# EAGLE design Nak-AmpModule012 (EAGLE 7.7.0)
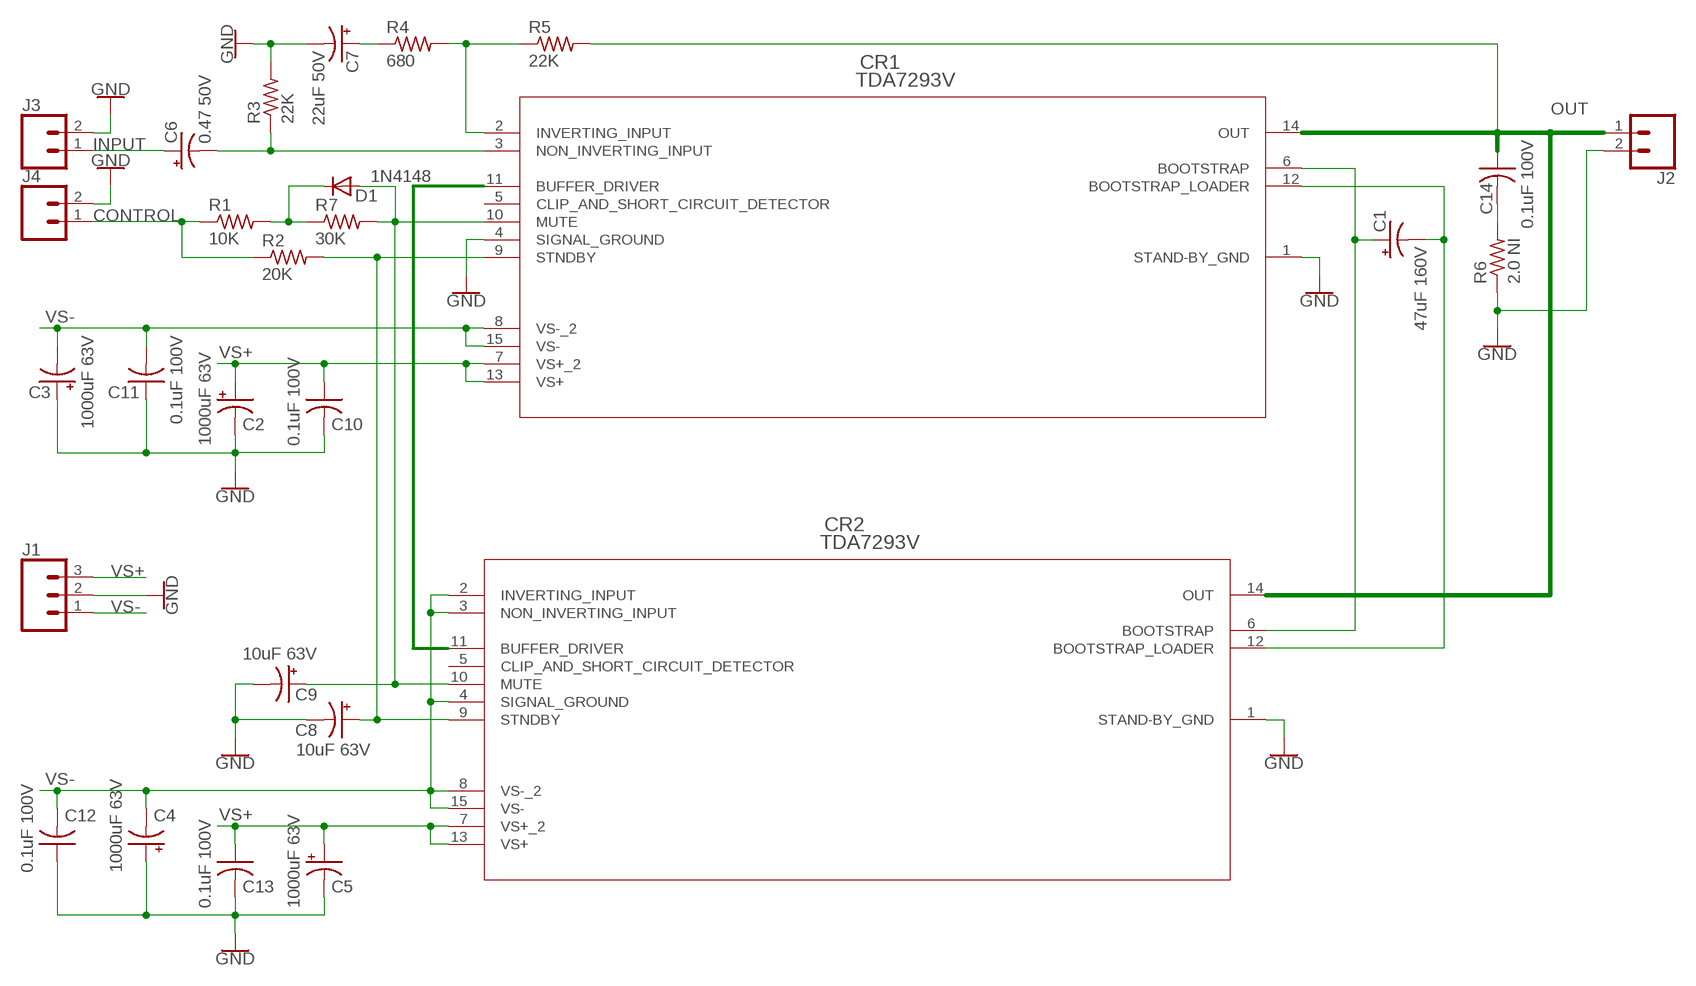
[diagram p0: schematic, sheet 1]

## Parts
C1  47uF 160V  CPOL-USE5-10.5  [E5-10,5]
C2  1000uF 63V  CPOL-USE7.5-16  [E7,5-16]
C3  1000uF 63V  CPOL-USE7.5-16  [E7,5-16]
C4  1000uF 63V  CPOL-USE7.5-16  [E7,5-16]
C5  1000uF 63V  CPOL-USE7.5-16  [E7,5-16]
C6  0.47 50V  CPOL-USE2-5  [E2-5]
C7  22uF 50V  CPOL-USE3.5-8  [E3,5-8]
C8  10uF 63V  CPOL-USE2.5-5  [E2,5-5]
C9  10uF 63V  CPOL-USE2.5-5  [E2,5-5]
C10  0.1uF 100V  C-US025-030X050  [C025-030X050]
C11  0.1uF 100V  C-US025-030X050  [C025-030X050]
C12  0.1uF 100V  C-US025-030X050  [C025-030X050]
C13  0.1uF 100V  C-US025-030X050  [C025-030X050]
C14  0.1uF 100V  C-US025-030X050  [C025-030X050]
CR1  TDA7293V  [MULTIWATT15_V]
CR2  TDA7293V  [MULTIWATT15_V]
D1  1N4148  1N4148DO35-7  [DO35-7]
J1  CONN_03-SCREW-5MM  [SCREWTERMINAL-5MM-3]
J2  CONN_025MM  [SCREWTERMINAL-5MM-2]
J3  CONN_023.5MM  [SCREWTERMINAL-3.5MM-2]
J4  CONN_023.5MM  [SCREWTERMINAL-3.5MM-2]
R1  10K  R-US_0207/10  [0207/10]
R2  20K  R-US_0207/10  [0207/10]
R3  22K  R-US_0204/7  [0204/7]
R4  680  R-US_0207/10  [0207/10]
R5  22K  R-US_0204/7  [0204/7]
R6  2.0 NI  R-US_0411/15  [0411/15]
R7  30K  R-US_0207/10  [0207/10]

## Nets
B-LOADER: C1.- CR1.12(BOOTSTRAP_LOADER) CR2.12(BOOTSTRAP_LOADER)
BOOTSTRAP: C1.+ CR1.6(BOOTSTRAP) CR2.6(BOOTSTRAP)
BUFDRVR: CR1.11(BUFFER_DRIVER) CR2.11(BUFFER_DRIVER)
CONTROL: J4.1 R1.1 R2.1
GND: C2.- C3.+ C4.+ C5.- C7.- C8.- C9.- C10.2 C11.1 C12.1 C13.2 CR1.1(STAND-BY_GND) CR1.4(SIGNAL_GROUND) CR2.1(STAND-BY_GND) J1.2 J2.2 J3.2 J4.2 R3.2 R6.1
INPUT: C6.+ J3.1
INV: CR1.2(INVERTING_INPUT) R4.2 R5.1
MUTE: C9.+ CR1.10(MUTE) CR2.10(MUTE) D1.A R7.2
N$3: C14.2 R6.2
N$11: D1.C R1.2 R7.1
N$16: C7.+ R4.1
NON-INV: C6.- CR1.3(NON_INVERTING_INPUT) R3.1
OUT: C14.1 CR1.14(OUT) CR2.14(OUT) J2.1 R5.2
STNDBY: C8.+ CR1.9(STNDBY) CR2.9(STNDBY) R2.2
VS+: C2.+ C5.+ C10.1 C13.1 CR1.7(VS+_2) CR1.13(VS+) CR2.7(VS+_2) CR2.13(VS+) J1.3
VS-: C3.- C4.- C11.2 C12.2 CR1.8(VS-_2) CR1.15(VS-) CR2.2(INVERTING_INPUT) CR2.3(NON_INVERTING_INPUT) CR2.4(SIGNAL_GROUND) CR2.8(VS-_2) CR2.15(VS-) J1.1
Unconnected: CR1.5(CLIP_AND_SHORT_CIRCUIT_DETECTOR) CR2.5(CLIP_AND_SHORT_CIRCUIT_DETECTOR)

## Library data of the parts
C1 = resistor:CPOL-US: POLARIZED CAPACITOR, American symbol; DESC: 47 µF 160 V Capacitor Radial, 10000 Hrs @ 105C; MFG: Rubycon; PN: 160BXC47MEFC10X20
C2 C3 C5-C9 = resistor:CPOL-US: POLARIZED CAPACITOR, American symbol
C4 = resistor:CPOL-US: POLARIZED CAPACITOR, American symbol; DESC: 1000 µF 63 V Electrolytic Capacitor Radial, 10000 Hrs @ 105°C; MFG: Rubycon; PN: 63ZLJ1000M16X25
C10 C12-C14 = resistor:C-US: CAPACITOR, American symbol
C11 = resistor:C-US: CAPACITOR, American symbol; DESC: 0.1 µF ±10% 100V Ceramic Capacitor X7R Radial; MFG: Vishay; PN: K104K20X7RH53L2
CR1 CR2 = STM-TDA7293V:TDA7293V; BUILT_BY: EMA_UL_Team; MANUFACTURER_PART_NUMBER: TDA7293V; VENDOR: STMicroelectronics
D1 = diode:1N4148: DIODE
J1 = SparkFun-Connectors:CONN_03: Multi connection point. Often used as Generic Header-pin footprint for 0.1 inch spaced/style header connections On any of the 0.1 inch spaced packages, you can populate with these: Break Away Headers - Straight (PRT-00116) Break Away Male Headers - Right Angle (PRT-00553) Female Headers (PRT-00115)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; PROD_ID: CONN-10134; SF_SKU: PRT-08433
J2 = SparkFun-Connectors:CONN_02: Multi connection point. Often used as Generic Header-pin footprint for 0.1 inch spaced/style header connections; SF_SKU: PRT-08432
J3 J4 = SparkFun-Connectors:CONN_02: Multi connection point. Often used as Generic Header-pin footprint for 0.1 inch spaced/style header connections; PROD_ID: CONN-08399
R1-R5 R7 = resistor:R-US_: RESISTOR, American symbol
R6 = resistor:R-US_: RESISTOR, American symbol; DESC: 2 Ohms ±1% 2W Resistor Axial Non-Inductive Wirewound; MFG: Ohmite; PN: WNC2R0FET

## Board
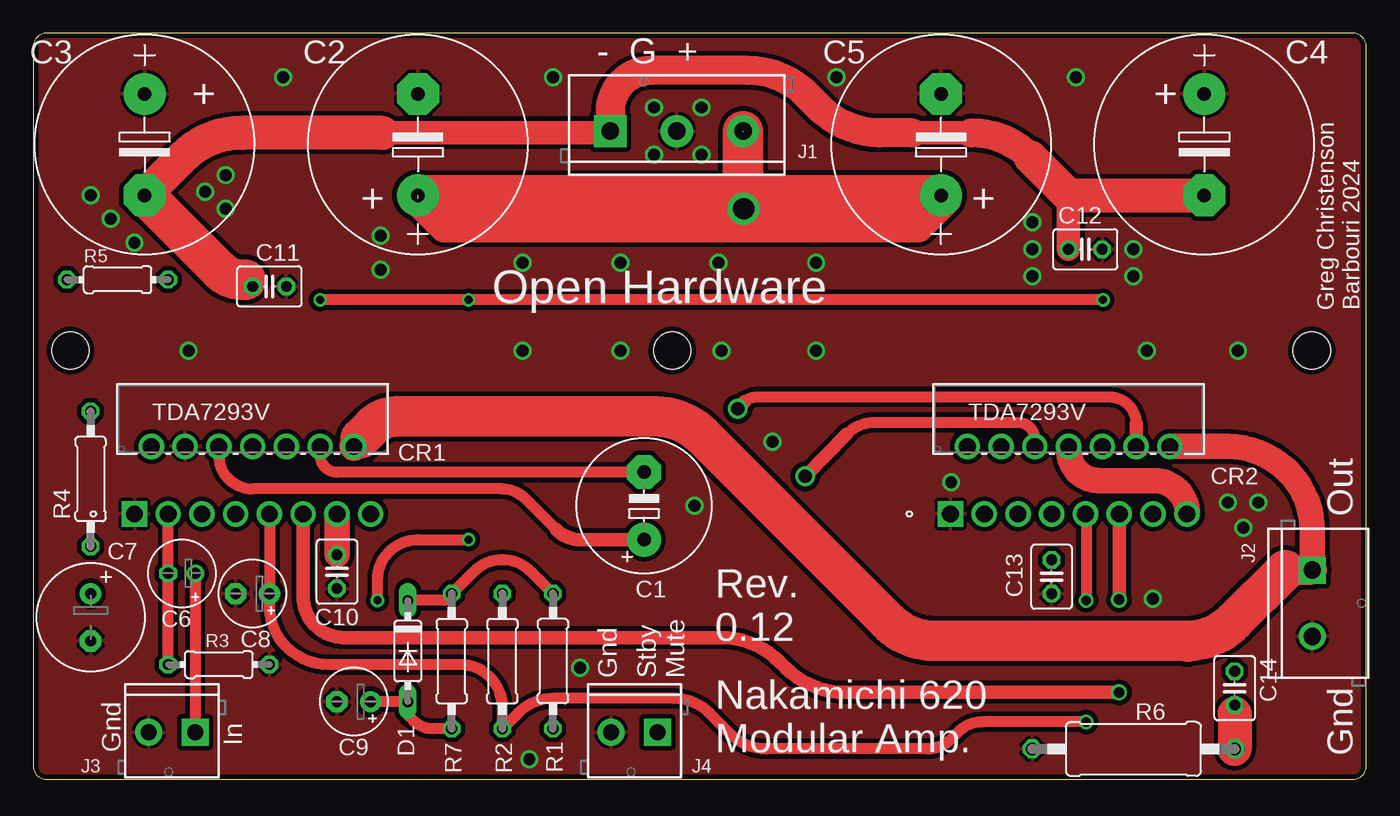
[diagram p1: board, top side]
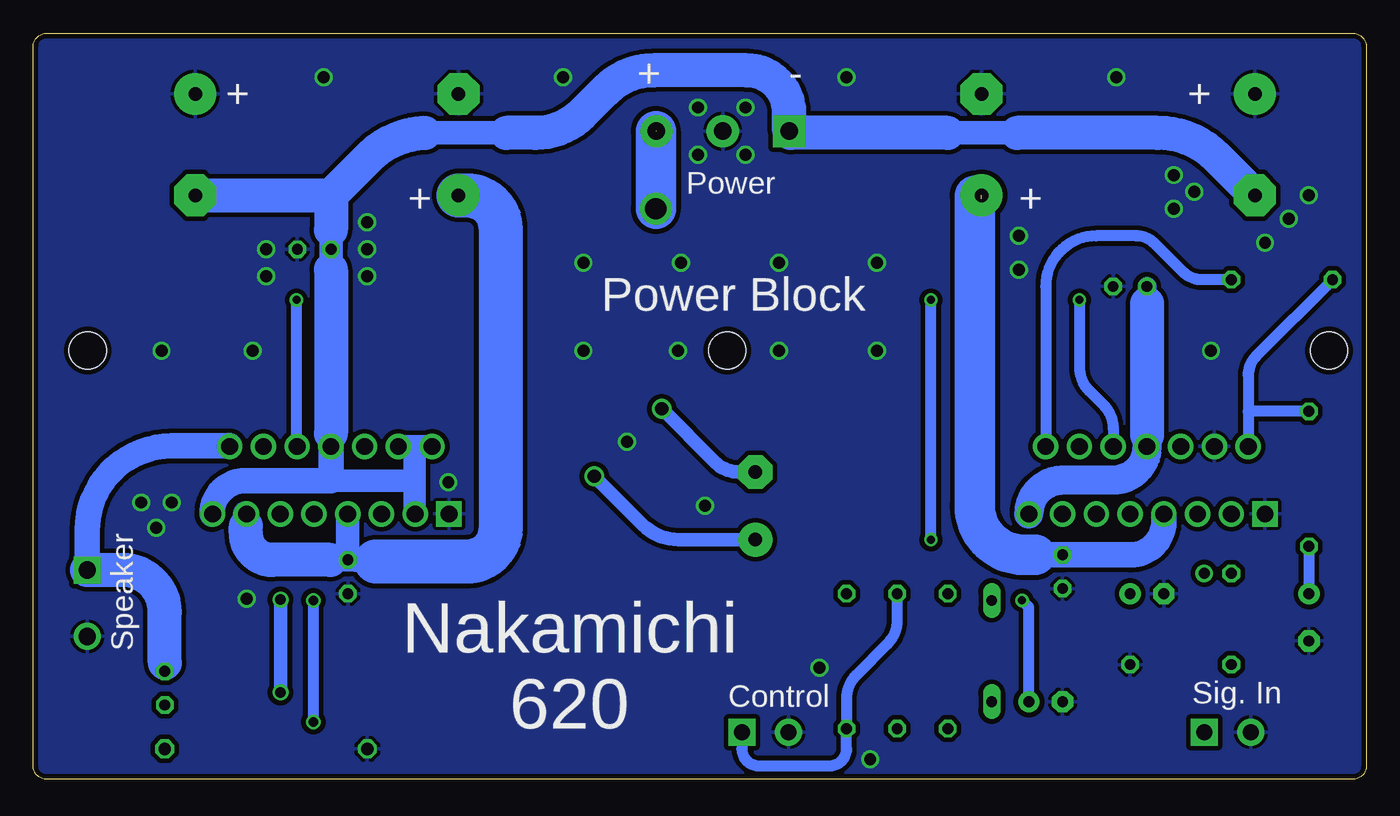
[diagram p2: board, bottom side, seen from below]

Size 100.33 x 56.13 mm. Coordinates in mm from the lower left corner, seen from the top.
Outline: 0,55.13 0,1 arc90 1,0 99.33,0 arc90 100.33,1 100.33,55.13 arc90 99.33,56.13 1,56.13 arc90 0,55.13
Copper layers (1*16): Top 0.035mm / dielectric 1.5mm / Bottom 0.035mm
Design rules "default *": minimum track width 14mil, minimum drill 9mil, track to track 14mil, track to pad 14mil, pad to pad 14mil, via to via 14mil, smd to smd 8mil, copper to edge 15mil, drill to drill 9mil, minimum pad ring 10mil, minimum via ring 8mil, stop-mask expansion 4mil, vias tented up to drill 24mil, thermal gap 10mil
Holes 2.8 mm at 2.79,32.26 48.11,32.26 96.23,32.26

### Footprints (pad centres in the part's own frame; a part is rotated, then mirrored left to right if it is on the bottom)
E5-10,5 = drill 1.016 pad 2.54: + -2.54,0 | drill 1.016 pad 2.54 octagon: - 2.54,0
E7,5-16 = drill 1.016 pad 3.15: + -3.81,0 | drill 1.016 pad 3.15 octagon: - 3.81,0
E2-5 = drill 0.813 pad 1.27: + -1.016,0 | drill 0.813 pad 1.27 octagon: - 1.016,0
E3,5-8 = drill 0.813 pad 1.6: + -1.778,0 | drill 0.813 pad 1.6 octagon: - 1.778,0
E2,5-5 = drill 0.813 pad 1.6: + -1.27,0 | drill 0.813 pad 1.6 octagon: - 1.27,0
C025-030X050 = drill 0.813 octagon: 1 -1.27,0; 2 1.27,0
MULTIWATT15_V = drill 1.27 pad 1.778 square: 1 -17.78,-14.326 | drill 1.27 pad 1.778: 2 -16.51,-9.246; 3 -15.24,-14.326; 4 -13.97,-9.246; 5 -12.7,-14.326; 6 -11.43,-9.246; 7 -10.16,-14.326; 8 -8.89,-9.246; 9 -7.62,-14.326; 10 -6.35,-9.246; 11 -5.08,-14.326; 12 -3.81,-9.246; 13 -2.54,-14.326; 14 -1.27,-9.246; 15 0,-14.326
DO35-7 = drill 0.813 long: A 3.81,0; C -3.81,0
SCREWTERMINAL-5MM-3 = drill 1.3 pad 2.413 square: 1 0,0 | drill 1.3 pad 2.413: 2 5,0; 3 10,0
SCREWTERMINAL-5MM-2 = drill 1.3 pad 2.032 square: 1 0,0 | drill 1.3 pad 2.032: 2 5,0
SCREWTERMINAL-3.5MM-2 = drill 1.2 pad 2.032 square: 1 0,0 | drill 1.2 pad 2.032: 2 3.5,0
0207/10 = drill 0.813 octagon: 1 -5.08,0; 2 5.08,0
0204/7 = drill 0.813 octagon: 1 -3.81,0; 2 3.81,0
0411/15 = drill 0.914 octagon: 1 -7.62,0; 2 7.62,0

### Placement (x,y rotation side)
C1  45.97,20.57 90 top
C2  28.96,47.75 90 top
C3  8.38,47.75 270 top
C4  88.14,47.75 270 top
C5  68.33,47.75 90 top
C6  11.18,15.49 180 top
C7  4.32,12.19 270 top
C8  16.51,13.97 180 top
C9  24.13,5.84 180 top
C10  22.86,15.62 270 top
C11  17.78,37.08 180 top
C12  79.18,39.88 180 top
C13  76.64,15.24 270 top
C14  90.42,6.86 270 top
CR1  25.4,34.29 0 top
CR2  86.82,34.29 0 top
D1  28.19,9.65 270 top
J1  43.43,48.77 0 top
J2  96.27,15.75 270 top
J3  12.19,3.56 180 top
J4  46.99,3.56 180 top
R1  39.12,8.89 90 top
R2  35.31,8.89 270 top
R3  13.97,8.64 0 top
R4  4.32,22.61 90 top
R5  6.35,37.59 0 top
R6  82.8,2.29 0 top
R7  31.5,8.89 270 top

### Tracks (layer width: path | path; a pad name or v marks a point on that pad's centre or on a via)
B-LOADER  (via drill 1)
  Top 0.813: CR1.12 21.59,24.38 arc90 22.86,23.11 C1.- | 53.54,28.39 arc-45 54.44,28.77 81.01,28.77 arc-90 83.01,26.77
  Top 1.016: v53.02,27.88 53.54,28.39 | 83.01,26.77 CR2.12
  Bottom 1.016: C1.- 47.21,23.11 arc45 49,23.86 v53.02,27.88
BOOTSTRAP  (via drill 1)
  Top 0.813: CR1.6 13.97,24.38 arc90 16.51,21.84 35.27,21.84 arc-45 37.07,21.1 39.39,18.78 | 61.21,25.97 arc-45 63.37,26.86 74.12,26.86 arc-90 75.39,25.59
  Top 1.016: C1.+ 41.18,18.03 arc-45 39.39,18.78 | v58.1,22.8 61.21,25.97 | 75.39,25.59 CR2.6
  Bottom 1.016: C1.+ 51.76,18.03 arc45 54.46,19.15 v58.1,22.8
BUFDRVR  (via drill 0.8)
  Top 0.813: 81.74,13.79 v81.72,13.53
  Top 1.016: CR2.11 81.74,13.79 | v81.72,6.54 61.11,6.54 arc-45 56.62,8.4 56.22,8.81 arc45 51.73,10.67 23.37,10.67 arc-90 20.32,13.72 CR1.11
  Bottom 1.016: v81.72,13.53 v81.72,6.54
CONTROL
  Bottom 0.813: R2.1 35.31,11.96 arc45 36.04,10.19 38.38,7.84 arc-45 39.12,6.08 R1.1 39.12,2.29 arc90 40.39,1.02 45.72,1.02 arc90 46.99,2.29 J4.1
GND  (via drill 0.9)
  other vias: 41.15,8.38 69.09,22.35 92.2,20.83 89.92,20.83 36.83,38.86 44.2,38.86 51.56,38.86 58.93,38.86 11.68,32.26 39.12,52.83 18.8,52.83 78.49,52.83 7.62,40.39 12.95,44.2 5.84,42.16 14.48,42.93 14.48,45.47 26.16,40.89 26.16,38.35 4.32,43.94 46.74,50.55 50.29,50.55 46.74,46.99 50.29,46.99 75.18,37.85 75.18,39.88 75.18,41.91 82.8,39.88 82.8,37.85 84.26,13.59 36.83,32.26 44.2,32.26 51.82,32.26 58.93,32.26 83.82,32.26 90.68,32.26 60.45,52.83 37.34,1.52 91.06,18.92 49.78,20.57 55.63,25.4
  pour Top: 0,0 100.33,0 100.33,56.13 0,56.13
  pour Bottom: 0,0 100.33,0 100.33,56.13 0,56.13
INPUT
  Top 0.813: C6.+ J3.1
INV
  Bottom 0.813: R4.2 8.89,27.69 | 8.89,27.69 CR1.2 | R5.1 8.3,31.83 arc-45 8.89,30.41 8.89,27.69
MUTE  (via drill 0.6)
  Top 0.813: v80.52,36.07 v32.77,36.07 v21.59,36.07 | R7.2 30.04,3.81 arc-45 28.62,4.4 28.19,4.83 D1.A C9.+ | v25.91,13.46 25.91,14.99 arc-90 28.96,18.03 v32.77,18.03
  Bottom 0.813: CR2.10 80.52,25.04 v80.52,36.07 | v21.59,36.07 21.59,31.02 arc-45 20.85,29.23 19.78,28.16 arc45 19.05,26.4 CR1.10 | C9.+ 25.4,12.95 v25.91,13.46 | v32.77,18.03 v32.77,36.07
N$3
  Top 1.27: C14.2 90.42,4.95
  Top 2.54: 90.42,4.95 R6.2
N$11
  Top 0.813: R1.2 37.46,15.62 arc90 33.15,15.62 R7.1 30.99,13.46 D1.C
N$16
  Bottom 0.813: R4.1 C7.+
NON-INV
  Top 0.813: CR1.3 C6.- R3.1
OUT
  Top 1.93: CR2.14 89.92,25.04 arc-90 96.27,18.69 J2.1
  Top 2.184: CR1.14 arc-45 24.2,25.22 24.64,25.65 | 94.23,15.75 J2.1 | 86.87,9.91 86.83,9.91 86.83,10.41
  Top 3.048: 24.64,25.65 25.55,26.56 arc-45 27.34,27.3 46.82,27.3 arc-45 50.36,25.84 64.32,11.88 arc45 67.86,10.41 86.83,10.41 arc45 90.36,11.88 94.23,15.75
  Bottom 0.813: R5.2 12.38,37.59 arc45 13.79,38.18 15.92,40.31 arc-45 17.34,40.89 20.32,40.89 arc-90 24.13,37.08 CR1.14
  Bottom 1.27: C14.1 90.42,8.76
  Bottom 1.93: J2.1 96.27,18.73 arc90 89.92,25.08 85.53,25.08
  Bottom 2.54: 90.42,8.76 90.42,12.57 arc-90 93.6,15.75 J2.1
STNDBY  (via drill 0.7)
  Top 0.813: CR2.9 79.25,19.96 v79.25,13.46 | v79.25,4.32 71.41,4.32 arc45 69.61,3.57 69.07,3.03 arc-45 67.27,2.29 55.17,2.29 arc-45 52.48,3.4 50.9,4.98 arc45 48.21,6.1 39.17,6.1 arc45 36.48,4.98 R2.2 35.31,5.46 arc90 32.13,8.64 22.23,8.64 arc-90 17.78,13.08 C8.+ CR1.9
  Bottom 0.813: v79.25,13.46 v79.25,4.32
VS+  (via drill 1.6)  (2 unrouted)
  Top 1.778: 53.34,43.94 53.43,43.94
  Top 1.93: CR1.13 C10.1
  Top 2.54: 68.58,43.69 66.55,41.66 30.99,41.66 28.96,43.69
  Top 3.048: C2.+ 53.34,43.94 | J1.3 53.43,43.94 C5.+
  Bottom 1.016: 84.33,19.96 CR2.13
  Bottom 1.778: 74.55,16.38 C13.1 | C13.1 76.66,16.51 CR2.7 | 77.98,16.51 C13.1
  Bottom 1.93: 84.33,19.96 84.33,19.05 | 24.89,16.89 C10.1 17.74,16.89 arc-90 15.24,19.39 CR1.7
  Bottom 2.54: 77.98,16.51 82.33,16.51 arc90 84.33,18.51 84.33,19.05
  Bottom 3.048: C2.+ 29.35,43.81 arc-45 29.46,43.92 29.46,20.57 arc-90 25.78,16.89 24.89,16.89 | 53.47,48.77 v53.47,42.93
  Bottom 3.302: C5.+ 67.69,43.94 arc90 65.15,41.4 65.15,18.92 arc90 67.69,16.38 74.55,16.38
VS-
  Top 1.016: 86.83,19.98 arc90 CR2.15 arc-90 86.83,19.98 | 86.87,19.98 86.83,19.98
  Top 1.676: C11.2 16,37.59
  Top 1.778: J1.1 43.31,48.64 26.29,48.64 | 77.92,43.94 C12.2 | 70.58,48.64 66.17,48.64
  Top 1.93: CR2.15 86.87,19.96 86.87,19.98 arc90 84.37,22.48 80.21,22.48 arc-90 77.93,24.77 CR2.8
  Top 2.184: 75.08,46.78 arc45 70.58,48.64 | J1.1 43.43,50.29 arc-90 46.48,53.34 53.76,53.34 arc-45 58.25,51.48 59.23,50.5 arc45 63.72,48.64 66.17,48.64
  Top 2.54: 26.29,48.64 15.71,48.64 arc45 11.22,46.78 C3.- | 75.08,46.78 77.92,43.94 C4.-
  Top 3.048: 16,37.59 15.77,37.59 arc-45 14,38.32 C3.-
  Bottom 1.016: 86.87,19.98 86.83,19.98 arc90 CR2.15
  Bottom 1.422: 77.92,43.94 77.92,44.07 | C11.2 16.51,35.81
  Bottom 1.676: CR2.2 71.63,25.04 | 71.63,25.04 CR2.4 | 71.63,19.96 71.63,22.48 | 71.63,22.48 71.63,25.04 | 77.92,22.48 71.63,22.48
  Bottom 1.778: 64.73,48.64 70.84,48.64 | CR2.3 71.63,19.96 | 77.92,38.35 C12.2 77.92,41.34 | 26.29,48.64 31.5,48.64
  Bottom 1.93: 77.92,26.04 77.92,25.06 CR2.8 | 86.87,19.94 86.87,19.98 arc90 84.37,22.48 77.92,22.48 77.92,25.02 | 16.51,25.91 CR1.8
  Bottom 2.184: CR1.8 arc90 19.05,22.5 22.86,22.5 arc-90 CR1.15
  Bottom 2.54: C3.- 11.22,46.78 arc-45 15.71,48.64 26.29,48.64 | 70.84,48.64 arc-45 75.33,46.53 77.92,43.94 | 77.92,38.35 77.92,26.04 | 16.51,35.81 16.51,25.91 | C4.- 77.92,43.94 | 31.5,48.64 43.31,48.64 J1.1 43.43,50.16 arc-90 46.61,53.34 53.68,53.34 arc-45 57.22,51.88 58.99,50.1 arc45 62.52,48.64 64.73,48.64 | 77.92,43.94 77.92,41.34

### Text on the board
tNames: - G + | + | + | + | + | Open Hardware | Greg Christenson / Barbouri 2024 | Out | Rev. / 0.12 | Gnd | Stby / Mute | In | Gnd | Nakamichi 620 / Modular Amp. | Gnd
bNames: - | + | + | + | Power | + | + | Power Block | Speaker | Sig. In | Control | Nakamichi / 620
